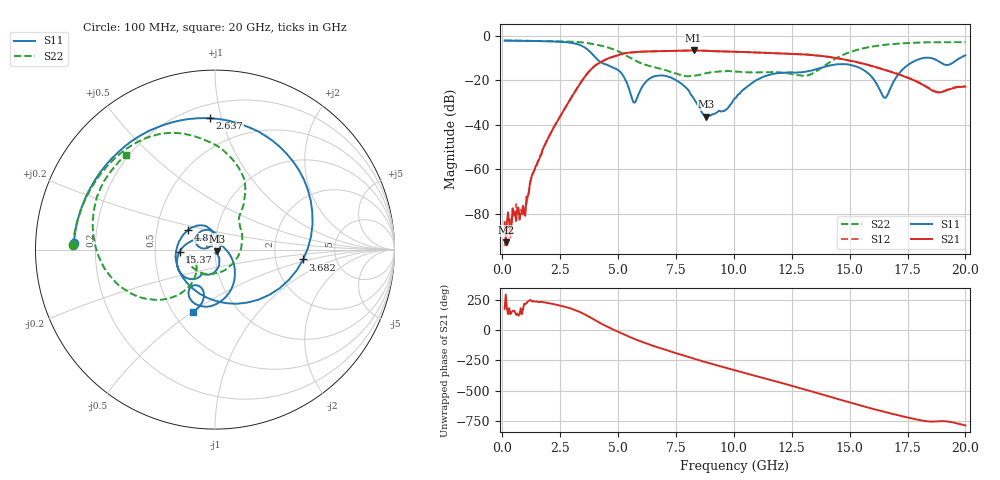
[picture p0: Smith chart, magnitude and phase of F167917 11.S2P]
!  2-Port S-parameters saved by WinCal
! VAR MeasName=S-Parameters (CALIBRATED_DATA) read from VNA (N5242A)
! VAR MeasDate=2016-11-22 9:00:13
! VAR NAME=F167917 11
! VAR FILENAME=F167917 11.S2P
! VAR DATE=2016-11-22 9:00:13
! VAR PHYS_PORTS=1,2
# Hz S DB R 50
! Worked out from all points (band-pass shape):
!   401 points, 100 MHz to 20 GHz, reference 50 ohm
!   highest |S21| = -6.50 dB at 8.259 GHz (marker M1); lowest = -92.8 dB at 149.8 MHz (marker M2)
!   |S21| within 3 dB of the highest: 4.744 GHz to 14.17 GHz (9.422 GHz wide, 99.7 % of centre)
!   lowest |S11| = -36.3 dB at 8.806 GHz (marker M3), VSWR 1.03, Z = 51.2 - j0.965 ohm
!   |S11| at or under -10 dB: 4.052 GHz to 18.15 GHz (14.1 GHz wide, 127 % of centre); 18.54 GHz to 19.75 GHz (1.212 GHz wide, 6.33 % of centre)
!   |S22| runs from -18.2 to -2.0 dB; largest |S21 - S12| = 0.0036
!   S11 on the Smith chart (normalised r, x): 100 MHz: 0.12, +0.02; 2.637 GHz: 0.29, +0.92; 3.682 GHz: 2.89, -0.42; 4.876 GHz: 0.73, +0.17; 15.37 GHz: 0.67, -0.02; 20 GHz: 0.63, -0.50
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1e8  -2.09 177.3  -83.85 176.3  -94.63 -176.2  -2.02 178.3
1.4975e8  -2.09 176.0  -92.84 -65.0  -92.18 83.5  -2.03 177.5
8.96e8  -2.20 156.1  -76.41 174.5  -81.12 -146.9  -2.15 165.7
1.3935e9  -2.28 141.8  -60.36 -124.2  -60.05 -126.2  -2.23 157.8
2.63725e9  -2.71 92.2  -33.72 -163.1  -33.75 -163.6  -2.47 135.6
3.43325e9  -4.45 27.0  -20.27 143.2  -20.30 143.2  -2.89 116.8
3.682e9  -6.12 -6.4  -16.79 118.4  -16.77 118.5  -3.20 109.9
4.08e9  -10.31 -78.2  -12.86 74.7  -12.82 74.6  -3.97 98.8
4.876e9  -14.68 143.4  -9.06 -2.4  -9.04 -2.6  -6.32 75.1
5.72175e9  -29.99 142.0  -7.27 -73.5  -7.27 -73.6  -10.93 56.8
6.7665e9  -17.82 139.2  -6.83 -145.2  -6.84 -145.4  -14.60 40.5
8.259e9  -28.12 36.9  -6.50 125.5  -6.52 125.6  -17.87 -70.1
8.80625e9  -36.27 -37.8  -6.70 94.3  -6.70 94.2  -16.70 -111.5
1.005e10  -28.08 -64.2  -7.10 27.9  -7.11 28.1  -16.00 -158.4
1.189075e10  -16.76 -106.0  -7.83 -67.5  -7.78 -67.4  -16.30 -166.7
1.338325e10  -15.47 -119.1  -8.59 -147.7  -8.55 -147.4  -16.99 -136.3
1.537325e10  -14.08 -176.7  -11.93 102.5  -11.94 102.3  -6.11 -147.6
1.646775e10  -27.58 76.7  -15.16 46.2  -15.08 46.8  -4.05 -171.1
1.67165e10  -24.59 2.9  -15.87 34.3  -15.90 35.0  -3.78 -176.0
1.7811e10  -11.26 -78.2  -20.10 -15.4  -19.94 -14.9  -3.05 164.6
1.8806e10  -11.16 -122.2  -25.43 -34.5  -25.22 -33.9  -2.78 148.9
2e10  -8.71 -109.8  -22.82 -68.1  -22.60 -68.2  -2.79 133.1
